
DATA_BLOCK DB3484
TITLE=
VERSION : 0.1

STRUCT
   CM_ID : STRING  [8 ] := '=PRM'; //COMPOSITE MACHINE
   STATION_ID : STRING  [8 ] := '++OP10'; //STATION - TRATTO - ZONE
   ELEMENT_ID : STRING  [8 ] := '+81FIL63'; //ELEMENT
   DB_ID : INT := 0 ; //DB SIZE OR TYPE
   PART_STYLE : STRING  [12 ]; //PART STYLE ON LAST STATION
   ACT_CYCLE_TIME : INT ; //ACTUAL CYCLE TIME FOR THIS STYLE
   COUNT_GOOD : INT ; //COUNTER GOOD PIECES
   COUNT_SCRAP : INT ; //COUNTER SCRAP PIECES
   SPARE_00 : ARRAY  [0 .. 15 ] OF //SPARE INTEGER
   INT ;
   SPARE_01 : ARRAY  [0 .. 17 ] OF //SPARE INTEGER
   INT ;
   CODE_EVENT : ARRAY  [0 .. 7 ] OF //CODE EVENT - EXTENDED FAULT CODE DIAGNOSTIC
   INT ;
   EVENT : STRUCT
E0000 : BOOL ; //+81FIL63-B21; MS. G81_FIL63_B21;58
E0001 : BOOL ; //+81FIL63-B21; ME. G81_FIL63_B21;01
E0002 : BOOL ; //+81FIL63-B22; MS. G81_FIL63_B22;58
E0003 : BOOL ; //+81FIL63-B22; ME. G81_FIL63_B22;01
E0004 : BOOL ; //+81FIL63-B22_1; MS. G81_FIL63_B22_1;58
E0005 : BOOL ; //+81FIL63-B22_1; ME. G81_FIL63_B22_1;01
E0006 : BOOL ;
E0007 : BOOL ;
E0008 : BOOL ;
E0009 : BOOL ;
E0010 : BOOL ;
E0011 : BOOL ;
E0012 : BOOL ;
E0013 : BOOL ;
E0014 : BOOL ;
E0015 : BOOL ;
E0016 : BOOL ;
E0017 : BOOL ;
E0018 : BOOL ;
E0019 : BOOL ;
E0020 : BOOL ;
E0021 : BOOL ;
E0022 : BOOL ;
E0023 : BOOL ;
E0024 : BOOL ;
E0025 : BOOL ;
E0026 : BOOL ;
E0027 : BOOL ;
E0028 : BOOL ;
E0029 : BOOL ;
E0030 : BOOL ;
E0031 : BOOL ;
E0032 : BOOL ; //+81FIL63-Y1;MS.GENERALI ERRORE;1
E0033 : BOOL ; //+81FIL63-Y1;MS.GENERALI AVVERTIMENTO;2
E0034 : BOOL ; //+81FIL63-Y1;MS.MODALITA MANUALE;16
E0035 : BOOL ; //+81FIL63-Y1;MS.MODO AUTOMATICO;19
E0036 : BOOL ; //+81FIL63-Y1;MS.RILASCIO;17
E0037 : BOOL ; //+81FIL63-Y1; MS. APERTO;58
E0038 : BOOL ; //+81FIL63-Y1; MS. VICINO;58
E0039 : BOOL ; //+81FIL63-Y1; MS. MS_07;58
E0040 : BOOL ; //+81FIL63-Y1; MS. MS_10;58
E0041 : BOOL ; //+81FIL63-Y1; MS. MS_11;58
E0042 : BOOL ; //+81FIL63-Y1; MS. MS_12;58
E0043 : BOOL ; //+81FIL63-Y1; MS. MS_13;58
E0044 : BOOL ; //+81FIL63-Y1; MS. MS_14;58
E0045 : BOOL ; //+81FIL63-Y1; MS. MS_15;58
E0046 : BOOL ; //+81FIL63-Y1; MS. MS_16;58
E0047 : BOOL ; //+81FIL63-Y1; MS. MS_17;58
E0048 : BOOL ; //+81FIL63-Y1; ME. ME_00;58
E0049 : BOOL ; //+81FIL63-Y1; ME. ME_01;58
E0050 : BOOL ; //+81FIL63-Y1; ME. ME_02;58
E0051 : BOOL ; //+81FIL63-Y1; ME. ME_03;58
E0052 : BOOL ; //+81FIL63-Y1; ME. ME_04;58
E0053 : BOOL ; //+81FIL63-Y1; ME. ME_05;58
E0054 : BOOL ; //+81FIL63-Y1; ME. ME_06;58
E0055 : BOOL ; //+81FIL63-Y1; ME. ME_07;58
E0056 : BOOL ; //+81FIL63-Y1; ME. ME_10;58
E0057 : BOOL ; //+81FIL63-Y1; ME. ME_11;58
E0058 : BOOL ; //+81FIL63-Y1; ME. ME_12;58
E0059 : BOOL ; //+81FIL63-Y1; ME. ME_13;58
E0060 : BOOL ; //+81FIL63-Y1; ME. ME_14;58
E0061 : BOOL ; //+81FIL63-Y1; ME. ME_15;58
E0062 : BOOL ; //+81FIL63-Y1; ME. ME_16;58
E0063 : BOOL ; //+81FIL63-Y1; ME. ME_17;58
END_STRUCT;
END_STRUCT;
BEGIN
CM_ID := '=PRM';
STATION_ID := '++OP10';
ELEMENT_ID := '+81FIL63';
DB_ID := 0 ;
PART_STYLE := '';
ACT_CYCLE_TIME := 0;
COUNT_GOOD := 0;
COUNT_SCRAP := 0;
SPARE_00[0] := 0;
SPARE_00[1] := 0;
SPARE_00[2] := 0;
SPARE_00[3] := 0;
SPARE_00[4] := 0;
SPARE_00[5] := 0;
SPARE_00[6] := 0;
SPARE_00[7] := 0;
SPARE_00[8] := 0;
SPARE_00[9] := 0;
SPARE_00[10] := 0;
SPARE_00[11] := 0;
SPARE_00[12] := 0;
SPARE_00[13] := 0;
SPARE_00[14] := 0;
SPARE_00[15] := 0;
SPARE_01[0] := 0;
SPARE_01[1] := 0;
SPARE_01[2] := 0;
SPARE_01[3] := 0;
SPARE_01[4] := 0;
SPARE_01[5] := 0;
SPARE_01[6] := 0;
SPARE_01[7] := 0;
SPARE_01[8] := 0;
SPARE_01[9] := 0;
SPARE_01[10] := 0;
SPARE_01[11] := 0;
SPARE_01[12] := 0;
SPARE_01[13] := 0;
SPARE_01[14] := 0;
SPARE_01[15] := 0;
SPARE_01[16] := 0;
SPARE_01[17] := 0;
CODE_EVENT[0] := 0;
CODE_EVENT[1] := 0;
CODE_EVENT[2] := 0;
CODE_EVENT[3] := 0;
CODE_EVENT[4] := 0;
CODE_EVENT[5] := 0;
CODE_EVENT[6] := 0;
CODE_EVENT[7] := 0;
EVENT.E0000 := FALSE;
EVENT.E0001 := FALSE;
EVENT.E0002 := FALSE;
EVENT.E0003 := FALSE;
EVENT.E0004 := FALSE;
EVENT.E0005 := FALSE;
EVENT.E0006 := FALSE;
EVENT.E0007 := FALSE;
EVENT.E0008 := FALSE;
EVENT.E0009 := FALSE;
EVENT.E0010 := FALSE;
EVENT.E0011 := FALSE;
EVENT.E0012 := FALSE;
EVENT.E0013 := FALSE;
EVENT.E0014 := FALSE;
EVENT.E0015 := FALSE;
EVENT.E0016 := FALSE;
EVENT.E0017 := FALSE;
EVENT.E0018 := FALSE;
EVENT.E0019 := FALSE;
EVENT.E0020 := FALSE;
EVENT.E0021 := FALSE;
EVENT.E0022 := FALSE;
EVENT.E0023 := FALSE;
EVENT.E0024 := FALSE;
EVENT.E0025 := FALSE;
EVENT.E0026 := FALSE;
EVENT.E0027 := FALSE;
EVENT.E0028 := FALSE;
EVENT.E0029 := FALSE;
EVENT.E0030 := FALSE;
EVENT.E0031 := FALSE;
EVENT.E0032 := FALSE;
EVENT.E0033 := FALSE;
EVENT.E0034 := FALSE;
EVENT.E0035 := FALSE;
EVENT.E0036 := FALSE;
EVENT.E0037 := FALSE;
EVENT.E0038 := FALSE;
EVENT.E0039 := FALSE;
EVENT.E0040 := FALSE;
EVENT.E0041 := FALSE;
EVENT.E0042 := FALSE;
EVENT.E0043 := FALSE;
EVENT.E0044 := FALSE;
EVENT.E0045 := FALSE;
EVENT.E0046 := FALSE;
EVENT.E0047 := FALSE;
EVENT.E0048 := FALSE;
EVENT.E0049 := FALSE;
EVENT.E0050 := FALSE;
EVENT.E0051 := FALSE;
EVENT.E0052 := FALSE;
EVENT.E0053 := FALSE;
EVENT.E0054 := FALSE;
EVENT.E0055 := FALSE;
EVENT.E0056 := FALSE;
EVENT.E0057 := FALSE;
EVENT.E0058 := FALSE;
EVENT.E0059 := FALSE;
EVENT.E0060 := FALSE;
EVENT.E0061 := FALSE;
EVENT.E0062 := FALSE;
EVENT.E0063 := FALSE;
END_DATA_BLOCK
